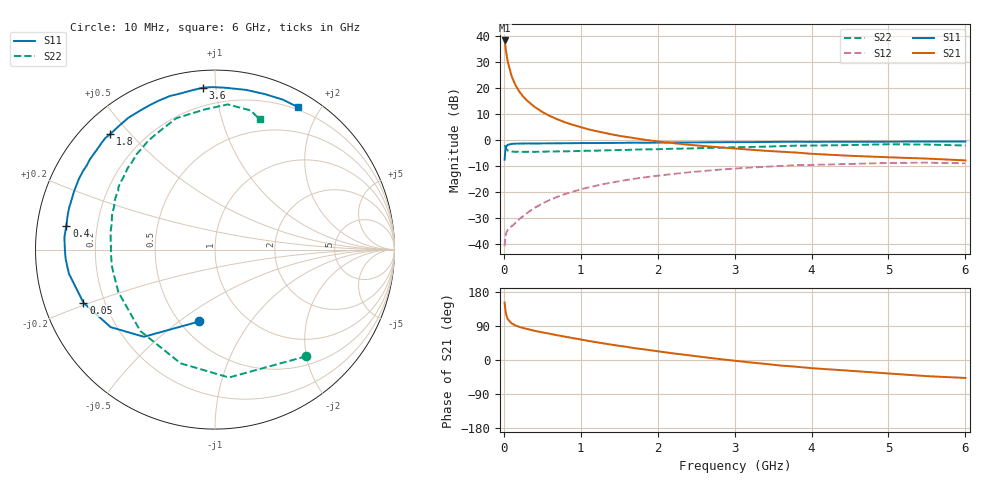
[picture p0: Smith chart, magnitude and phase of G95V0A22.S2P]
! SIEMENS Small Signal Semiconductors
! BFG235
! Si NPN RF Bipolar Junction Transistor in SOT223
! VCE = 5 V  IC = 220 mA
! Common Emitter S-Parameters:  July  1994
# GHz  S  MA  R  50
!  f  S11  S21  S12  S22
! GHz  MAG  ANG  MAG  ANG  MAG  ANG  MAG  ANG
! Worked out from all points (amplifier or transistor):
!   40 points, 10 MHz to 6 GHz, reference 50 ohm
!   highest |S21| = 38.1 dB at 10 MHz (marker M1)
!   |S21| within 3 dB of that: start of sweep to 23.54 MHz
!   unconditionally stable (mu >= 1): 420.9 MHz to 1.544 GHz
!   at 200 MHz: K = 0.84, MSG = 24.6 dB, |S12| = -30.7 dB
!   at 1.5 GHz: K = 1.01, MAG = 8.2 dB, |S12| = -16.0 dB
!   at 6 GHz: K = 0.90, MSG = 0.6 dB, |S12| = -9.1 dB
!   S11 on the Smith chart (normalised r, x): 10 MHz: 0.62, -0.60; 50 MHz: 0.12, -0.19; 400 MHz: 0.09, +0.08; 1.8 GHz: 0.08, +0.44; 3.6 GHz: 0.09, +0.92; 6 GHz: 0.17, +1.72
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0.01  0.4096 -102.3  80.44 151.3  0.0089 59.5  0.7825 -49.4
0.02  0.6267 -129.2  62.31 131.8  0.0134 45.6  0.7168 -83.8
0.03  0.7245 -143.4  48.31 120.1  0.0158 40.4  0.662 -106.8
0.05  0.7904 -158.0  31.83 108.1  0.0183 34.6  0.6155 -132.5
0.1  0.8251 -170.7  16.73 96.8  0.0213 39.1  0.5883 -156.2
0.15  0.8339 -176.5  11.21 91.1  0.0249 47.0  0.5804 -166.0
0.2  0.836 -179.6  8.389 87.6  0.0293 51.1  0.5822 -171.3
0.25  0.8387 177.5  6.749 84.4  0.0338 54.3  0.5797 -174.9
0.3  0.8419 175.2  5.638 82.0  0.0384 57.8  0.5804 -178.0
0.4  0.8386 170.8  4.242 77.0  0.0486 60.2  0.58 177.9
0.5  0.8424 167.4  3.387 72.9  0.0587 61.3  0.5843 174.5
0.6  0.8454 164.3  2.827 69.2  0.0691 61.2  0.5881 171.4
0.7  0.8459 160.8  2.438 65.0  0.0796 61.1  0.5916 168.6
0.9  0.851 155.3  1.913 57.7  0.0996 58.8  0.598 164.0
1.1  0.8558 149.1  1.572 50.3  0.1198 56.0  0.6086 159.1
1.8  0.8686 132.2  1.005 28.7  0.1845 43.6  0.6465 144.8
2.2  0.8788 123.4  0.853 17.5  0.2178 36.1  0.6658 136.9
3.2  0.8912 102.2  0.639 -6.3  0.2886 16.6  0.7189 118.3
3.6  0.9046 94.3  0.584 -14.7  0.3106 8.2  0.7459 110.1
4.5  0.9067 78.9  0.487 -28.4  0.3391 -7.9  0.7834 94.0
5.5  0.9169 65.7  0.43 -42.6  0.3591 -26.0  0.8005 75.7
6  0.9183 59.9  0.397 -47.4  0.3491 -32.8  0.768 71.1
